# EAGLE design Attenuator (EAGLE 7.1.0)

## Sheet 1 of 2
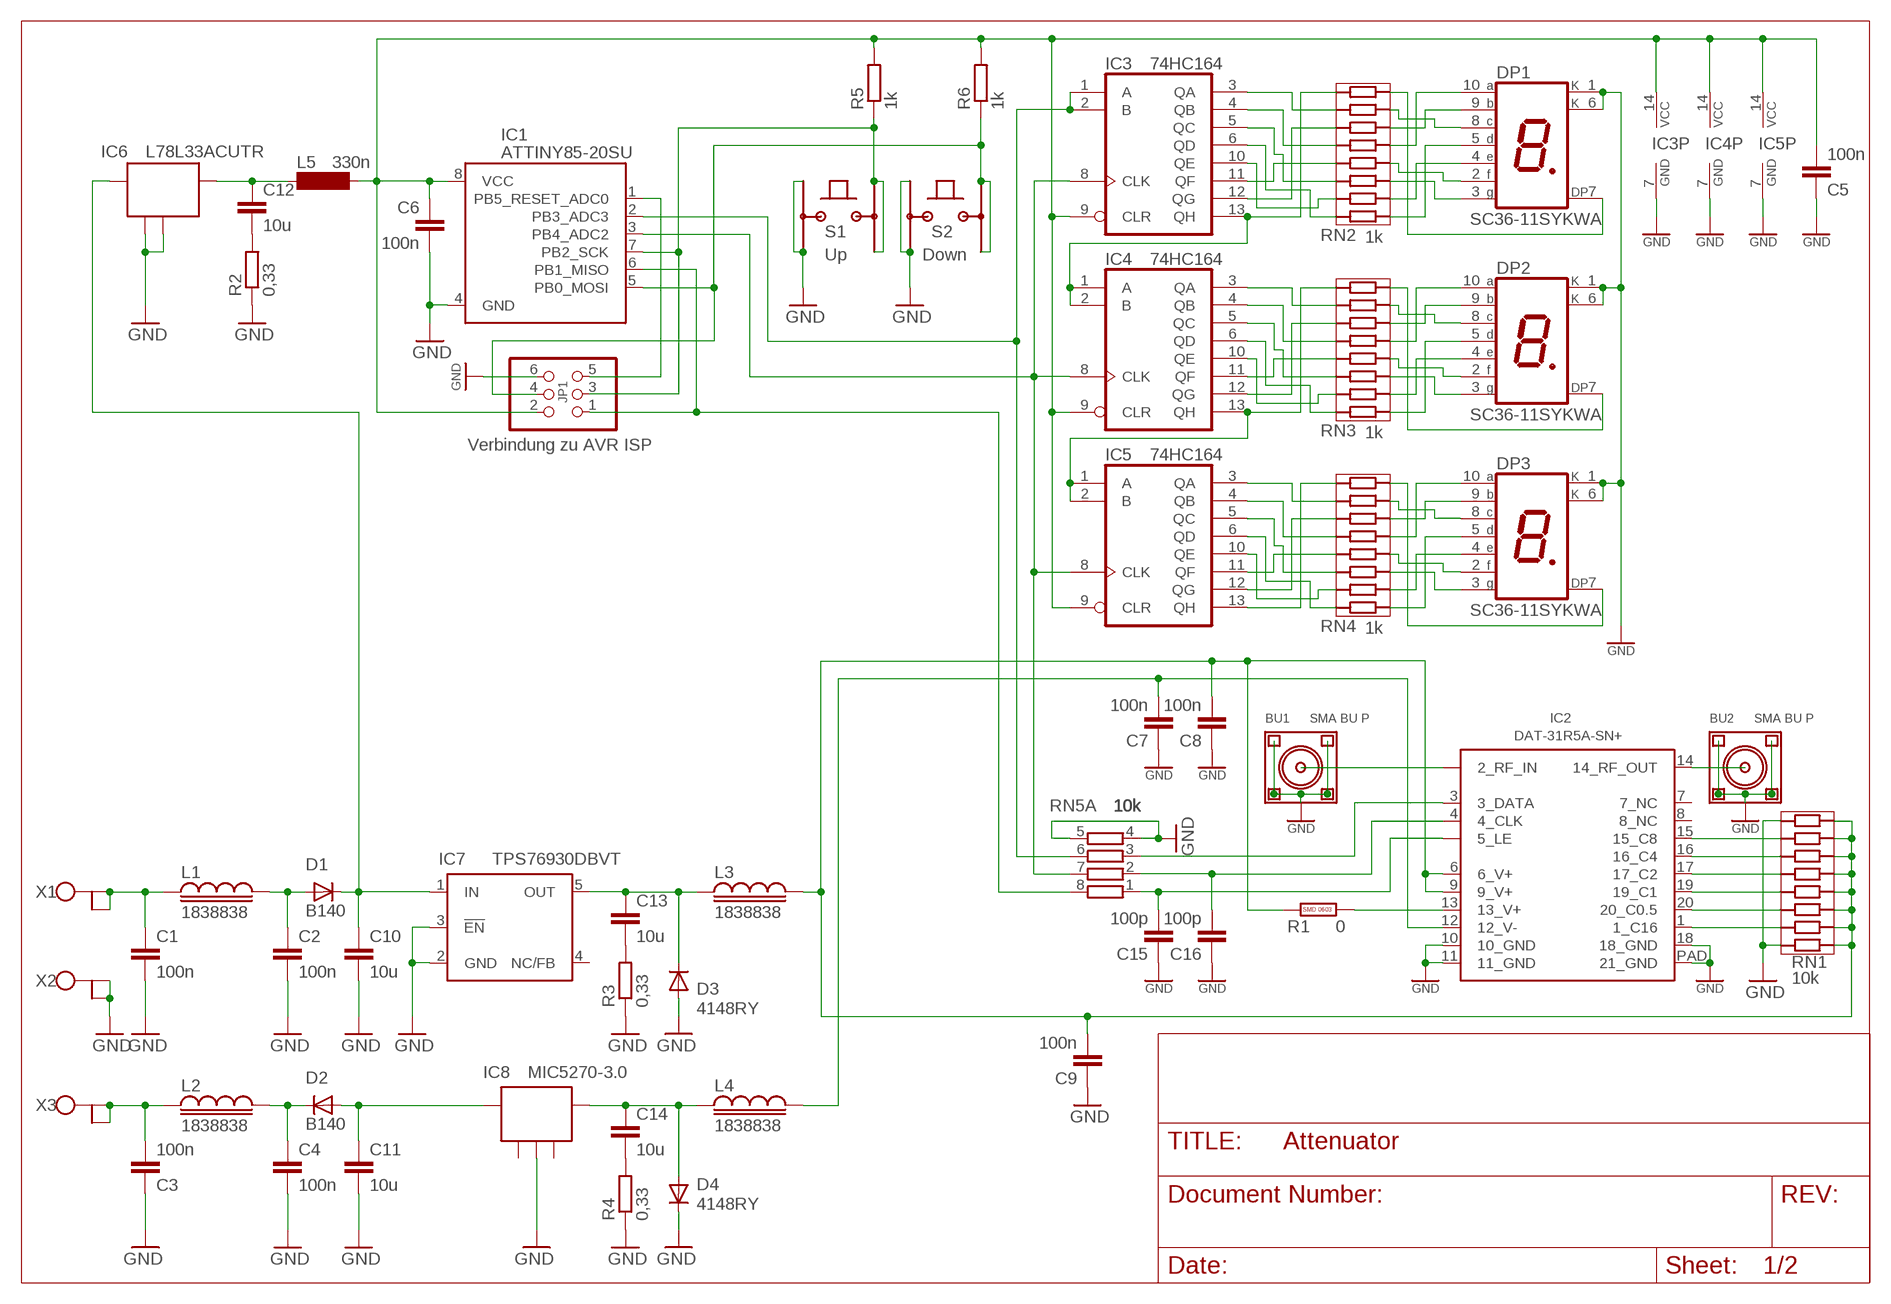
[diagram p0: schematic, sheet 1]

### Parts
BU1  SMA BU P  SMA_BUCHSE_STEHEND  [BU_SMA_STEHEND]
BU2  SMA BU P  SMA_BUCHSE_STEHEND  [BU_SMA_STEHEND]
C1  100n  C-EUC0805  [C0805]
C2  100n  C-EUC0805  [C0805]
C3  100n  C-EUC0805  [C0805]
C4  100n  C-EUC0805  [C0805]
C5  100n  C-EUC0805  [C0805]
C6  100n  C-EUC1206  [C1206]
C7  100n  C-EUC0603K  [C0603K]
C8  100n  C-EUC0603K  [C0603K]
C9  100n  C-EUC0603K  [C0603K]
C10  10u  C-EUC0805  [C0805]
C11  10u  C-EUC0805  [C0805]
C12  10u  C-EUC0805  [C0805]
C13  10u  C-EUC0805  [C0805]
C14  10u  C-EUC0805  [C0805]
C15  100p  C-EUC0603K  [C0603K]
C16  100p  C-EUC0603K  [C0603K]
D1  B140  DIODE-DO214AC  [DO214AC]
D2  B140  DIODE-DO214AC  [DO214AC]
D3  4148RY  TS4148_0805  [DIODE_0805]
D4  4148RY  TS4148_0805  [DIODE_0805]
DP1  SC36-11SYKWA  SC36-11SWRA_ROUND  [SC36-11SWRA_ROUND]
DP2  SC36-11SYKWA  SC36-11SWRA_ROUND  [SC36-11SWRA_ROUND]
DP3  SC36-11SYKWA  SC36-11SWRA_ROUND  [SC36-11SWRA_ROUND]
IC1  ATTINY85-20SU  [8S2]
IC2  DAT-31R5A-SN+  DAT-31-PP  [DG983-1]
IC3  74HC164  74AC164D  [SO14]
IC4  74HC164  74AC164D  [SO14]
IC5  74HC164  74AC164D  [SO14]
IC6  L78L33ACUTR  78XX_SOT89  [SOT89]
IC7  TPS76930DBVT  TPS77001  [SOT23-DBV]
IC8  MIC5270-3.0  [SOT23-5]
JP1  Verbindung zu AVR ISP  PINHD-2X3_2.54-SMD  [2X03SMD]
L1  1838838  L_0805  [SMD_0805]
L2  1838838  L_0805  [SMD_0805]
L3  1838838  L_0805  [SMD_0805]
L4  1838838  L_0805  [SMD_0805]
L5  330n  SM-1206  [SM-1206]
R1  0  MY_R0603  [X0603]
R2  0,33  R-EU_R0805  [R0805]
R3  0,33  R-EU_R0805  [R0805]
R4  0,33  R-EU_R0805  [R0805]
R5  1k  R-EU_R0805  [R0805]
R6  1k  R-EU_R0805  [R0805]
RN1  10k  RN_742C163  [RN_8_0.8MM]
RN2  1k  RN_742C163  [RN_8_0.8MM]
RN3  1k  RN_742C163  [RN_8_0.8MM]
RN4  1k  RN_742C163  [RN_8_0.8MM]
RN5  10k  4R-NEXB38V  [EXB38V]
S1  Up  TASTER9315  [TASTER9315]
S2  Down  TASTER9315  [TASTER9315]
X1  WAGO236-1  [WAGO236-1]
X2  WAGO236-1  [WAGO236-1]
X3  WAGO236-1  [WAGO236-1]

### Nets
+3,3V: C5.2 C6.1 IC1.8(VCC) IC3.9(CLR) IC3.14(VCC) IC4.9(CLR) IC4.14(VCC) IC5.9(CLR) IC5.14(VCC) JP1.2 L5.2 R5.2 R6.2
+3V: C8.2 C9.2 IC2.6(6_V+) IC2.9(9_V+) L3.2 R1.2 RN1.1 RN1.2 RN1.3 RN1.4 RN1.5 RN1.6 RN1.7 RN1.8
-3V: C7.2 IC2.12(12_V-) L4.2
CLK: IC1.3(PB4_ADC2) IC3.8(CLK) IC4.8(CLK) IC5.8(CLK) RN5.7
DATA: IC1.2(PB3_ADC3) IC3.1(A) IC3.2(B) RN5.6
GND: BU1.GND BU1.GND@1(GND) BU1.GND@2(GND) BU1.GND@3(GND) BU2.GND BU2.GND@1(GND) BU2.GND@2(GND) BU2.GND@3(GND) C1.2 C2.2 C3.1 C4.2 C5.1 C6.2 C7.1 C8.1 C9.1 C10.2 C11.2 C15.1 C16.1 D3.A D4.K(C) DP1.1(A) DP1.6(A) DP2.1(A) DP2.6(A) DP3.1(A) DP3.6(A) IC1.4(GND) IC2.10(10_GND) IC2.11(11_GND) IC2.18(18_GND) IC2.PAD(21_GND) IC3.7(GND) IC4.7(GND) IC5.7(GND) IC6.2(GND) IC6.2@1(CASE) IC7.2(GND) IC7.3(!EN) IC8.2(GND) JP1.6 R2.1 R3.1 R4.1 RN1.9 RN1.16 RN5.4 RN5.5 S1.1 S1.2 S2.1 S2.2 X2.1(KL) X2.2(KL1) ; also sheet 2
MISO: IC1.6(PB1_MISO) JP1.1 RN5.8
MOSI: IC1.5(PB0_MOSI) JP1.4 R6.1 S2.3 S2.4
N$1: IC2.3(3_DATA) RN5.3
N$2: C10.1 D1.C IC6.3(OUT) IC7.1(IN)
N$3: C1.1 L1.1 X1.1(KL) X1.2(KL1)
N$4: C12.2 R2.2
N$5: C2.1 D1.A L1.2
N$6: IC2.1(1_C16) RN1.10
N$7: C13.2 R3.2
N$9: IC2.20(20_C0.5) RN1.11
N$10: IC2.19(19_C1) RN1.12
N$11: IC2.17(17_C2) RN1.13
N$12: IC2.16(16_C4) RN1.14
N$13: IC2.15(15_C8) RN1.15
N$14: C16.2 IC2.4(4_CLK) RN5.2
N$15: C15.2 IC2.5(5_LE) RN5.1
N$16: IC2.13(13_V+) R1.1
N$19: C13.1 D3.K(C) IC7.5(OUT) L3.1
N$59: C14.2 R4.2
N$60: C12.1 IC6.1(IN) L5.1
N$61: C3.2 L2.1 X3.1(KL) X3.2(KL1)
N$62: C4.1 D2.C L2.2
N$63: C11.1 D2.A IC8.5(-IN)
N$64: C14.1 D4.A IC8.4(-OUT) L4.1
N$73: DP2.7(DP) RN3.16
N$80: DP2.8(C) RN3.15
N$81: DP2.9(B) RN3.14
N$82: DP2.10(A) RN3.13
N$83: DP2.2(F) RN3.12
N$84: DP2.3(G) RN3.11
N$85: DP2.4(E) RN3.10
N$86: DP2.5(D) RN3.9
N$87: DP1.7(DP) RN2.16
N$88: IC4.13(QH) IC5.1(A) IC5.2(B) RN3.1
N$89: IC4.5(QC) RN3.6
N$90: IC4.3(QA) RN3.2
N$91: IC4.12(QG) RN3.3
N$92: IC4.4(QB) RN3.4
N$93: IC4.11(QF) RN3.5
N$94: IC4.10(QE) RN3.7
N$96: IC4.6(QD) RN3.8
N$97: DP1.8(C) RN2.15
N$98: DP1.9(B) RN2.14
N$99: DP1.10(A) RN2.13
N$100: DP1.2(F) RN2.12
N$101: DP1.3(G) RN2.11
N$102: DP1.4(E) RN2.10
N$103: DP1.5(D) RN2.9
N$105: IC3.13(QH) IC4.1(A) IC4.2(B) RN2.1
N$106: IC3.3(QA) RN2.2
N$107: IC3.12(QG) RN2.3
N$108: IC3.4(QB) RN2.4
N$109: IC3.11(QF) RN2.5
N$110: IC3.5(QC) RN2.6
N$111: IC3.10(QE) RN2.7
N$112: IC3.6(QD) RN2.8
N$113: DP3.7(DP) RN4.16
N$114: DP3.8(C) RN4.15
N$115: DP3.9(B) RN4.14
N$116: DP3.10(A) RN4.13
N$117: DP3.2(F) RN4.12
N$118: DP3.3(G) RN4.11
N$119: DP3.4(E) RN4.10
N$120: DP3.5(D) RN4.9
N$122: IC5.13(QH) RN4.1
N$123: IC5.3(QA) RN4.2
N$124: IC5.12(QG) RN4.3
N$125: IC5.4(QB) RN4.4
N$126: IC5.11(QF) RN4.5
N$127: IC5.5(QC) RN4.6
N$128: IC5.10(QE) RN4.7
N$129: IC5.6(QD) RN4.8
RESET1: IC1.1(PB5_RESET_ADC0) JP1.5
RF_IN: BU1.SIGNAL IC2.2(2_RF_IN)
RF_OUT: BU2.SIGNAL IC2.14(14_RF_OUT)
SCK: IC1.7(PB2_SCK) JP1.3 R5.1 S1.3 S1.4
Unconnected: IC2.7(7_NC) IC2.8(8_NC) IC7.4(NC/FB) IC8.1(NC1) IC8.3(NC2)

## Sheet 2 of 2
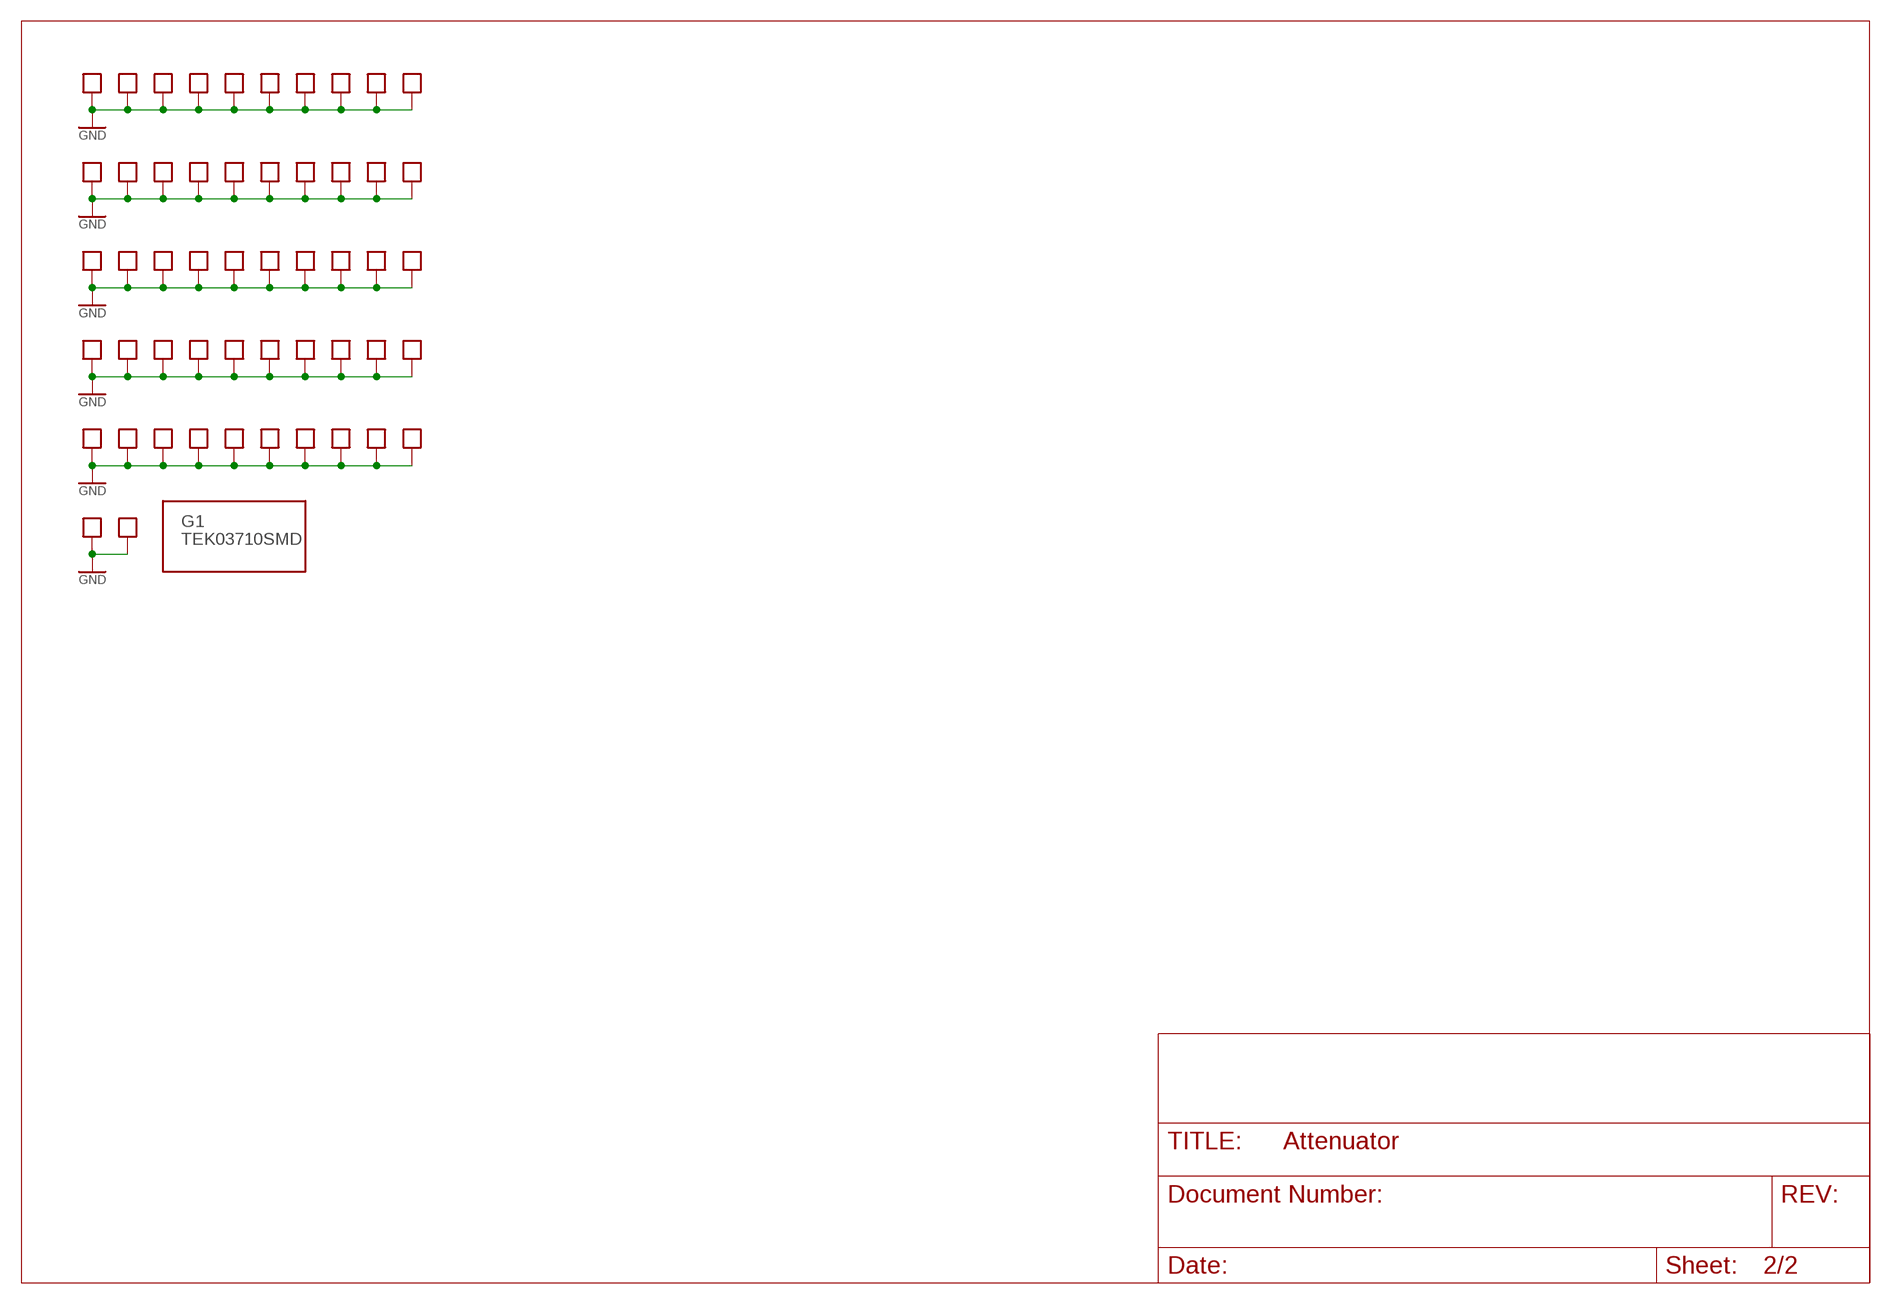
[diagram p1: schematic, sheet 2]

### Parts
G1  TEK03710SMD  [TEKO3710SMD]
GP1  PAD_1X1.5  [PAD_254X381]
GP2  PAD_1X1.5  [PAD_254X381]
GP3  PAD_1X1.5  [PAD_254X381]
GP4  PAD_1X1.5  [PAD_254X381]
GP5  PAD_1X1.5  [PAD_254X381]
GP6  PAD_1X1.5  [PAD_254X381]
GP7  PAD_1X1.5  [PAD_254X381]
GP8  PAD_1X1.5  [PAD_254X381]
GP9  PAD_1X1.5  [PAD_254X381]
GP10  PAD_1X1.5  [PAD_254X381]
GP11  PAD_1X1.5  [PAD_254X381]
GP12  PAD_1X1.5  [PAD_254X381]
GP13  PAD_1X1.5  [PAD_254X381]
GP14  PAD_1X1.5  [PAD_254X381]
GP15  PAD_1X1.5  [PAD_254X381]
GP16  PAD_1X1.5  [PAD_254X381]
GP17  PAD_1X1.5  [PAD_254X381]
GP18  PAD_1X1.5  [PAD_254X381]
GP19  PAD_1X1.5  [PAD_254X381]
GP20  PAD_1X1.5  [PAD_254X381]
GP21  PAD_1X1.5  [PAD_254X381]
GP22  PAD_1X1.5  [PAD_254X381]
GP23  PAD_1X1.5  [PAD_254X381]
GP24  PAD_1X1.5  [PAD_254X381]
GP25  PAD_1X1.5  [PAD_254X381]
GP26  PAD_1X1.5  [PAD_254X381]
GP27  PAD_1X1.5  [PAD_254X381]
GP28  PAD_1X1.5  [PAD_254X381]
GP29  PAD_1X1.5  [PAD_254X381]
GP30  PAD_1X1.5  [PAD_254X381]
GP31  PAD_1X1.5  [PAD_254X381]
GP32  PAD_1X1.5  [PAD_254X381]
GP33  PAD_1X1.5  [PAD_254X381]
GP34  PAD_1X1.5  [PAD_254X381]
GP35  PAD_1X1.5  [PAD_254X381]
GP36  PAD_1X1.5  [PAD_254X381]
GP37  PAD_1X1.5  [PAD_254X381]
GP38  PAD_1X1.5  [PAD_254X381]
GP39  PAD_1X1.5  [PAD_254X381]
GP40  PAD_1X1.5  [PAD_254X381]
GP41  PAD_1X05  [PAD_254X127]
GP42  PAD_1X1.5  [PAD_254X381]
GP43  PAD_1X1.5  [PAD_254X381]
GP44  PAD_1X1.5  [PAD_254X381]
GP45  PAD_1X1.5  [PAD_254X381]
GP46  PAD_1X1.5  [PAD_254X381]
GP47  PAD_1X1.5  [PAD_254X381]
GP48  PAD_1X1.5  [PAD_254X381]
GP49  PAD_1X1.5  [PAD_254X381]
GP50  PAD_1X1.5  [PAD_254X381]
GP51  PAD_1X1.5  [PAD_254X381]
GP52  PAD_1X05  [PAD_254X127]

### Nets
GND: GP1.TP(GND) GP2.TP(GND) GP3.TP(GND) GP4.TP(GND) GP5.TP(GND) GP6.TP(GND) GP7.TP(GND) GP8.TP(GND) GP9.TP(GND) GP10.TP(GND) GP11.TP(GND) GP12.TP(GND) GP13.TP(GND) GP14.TP(GND) GP15.TP(GND) GP16.TP(GND) GP17.TP(GND) GP18.TP(GND) GP19.TP(GND) GP20.TP(GND) GP21.TP(GND) GP22.TP(GND) GP23.TP(GND) GP24.TP(GND) GP25.TP(GND) GP26.TP(GND) GP27.TP(GND) GP28.TP(GND) GP29.TP(GND) GP30.TP(GND) GP31.TP(GND) GP32.TP(GND) GP33.TP(GND) GP34.TP(GND) GP35.TP(GND) GP36.TP(GND) GP37.TP(GND) GP38.TP(GND) GP39.TP(GND) GP40.TP(GND) GP41.TP(GND) GP42.TP(GND) GP43.TP(GND) GP44.TP(GND) GP45.TP(GND) GP46.TP(GND) GP47.TP(GND) GP48.TP(GND) GP49.TP(GND) GP50.TP(GND) GP51.TP(GND) GP52.TP(GND) ; also sheet 1

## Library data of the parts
BU1 BU2 = Diverse Analog:SMA_BUCHSE_STEHEND
C1-C16 = rcl:C-EU: CAPACITOR, European symbol
D1 D2 = diode:DIODE-: DIODE
D3 D4 = Dioden:TS4148_0805
DP1-DP3 = Displays:SC36-11SWRA_ROUND
G1 = Diverse Analog:TEK03710SMD
GP1-GP40 GP42-GP51 = Diverse Analog:PAD_1X1.5
GP41 GP52 = Diverse Analog:PAD_1X05
IC1 = Diverse Analog:ATTINY85-20SU
IC2 = Diverse Analog:DAT-31-PP
IC3-IC5 = 74xx-eu:74*164: 8-bit parallel out SHIFT REGISTER
IC6 = Diverse Analog:78XX_SOT89
IC7 = texas:TPS770*: ULTRALOW-POWER 50-mA LOW-DROPOUT LINEAR REGULATORS 50-mA Low-Dropout Regulator Source: http://focus.ti.com/lit/ds/symlink/tps77001.pdf
IC8 = Diverse Analog:MIC5270-3.0
JP1 = pinhead1:PINHD-2X3: PIN HEADER
L1-L4 = Diverse Analog:L_0805
L5 = inductor-neosid:SM-1206: INDUCTOR
R1 = Diverse Analog:MY_R0603
R2-R6 = rcl:R-EU_: RESISTOR, European symbol
RN1-RN4 = Diverse Analog:RN_742C163
RN5 = resistor-dil:4R-N: Array Chip Resistor Source: RS Component / Phycomp
S1 S2 = Diverse Analog:TASTER9315
X1-X3 = Diverse Analog:WAGO236-1

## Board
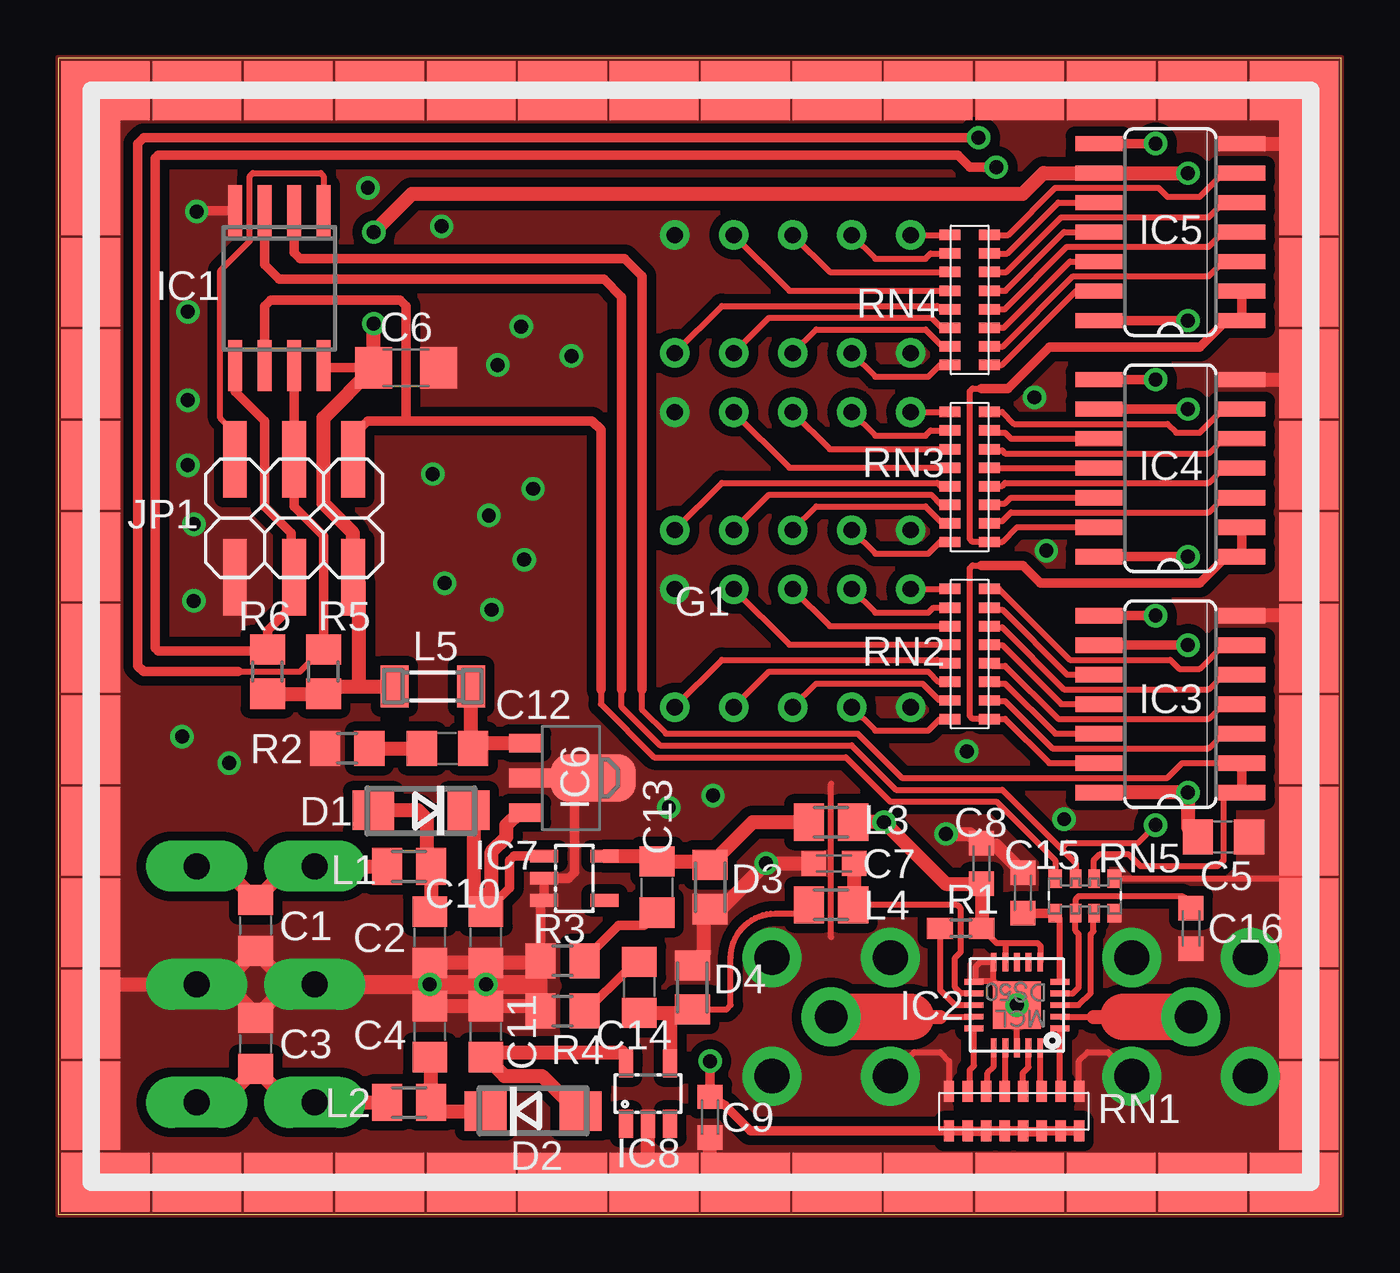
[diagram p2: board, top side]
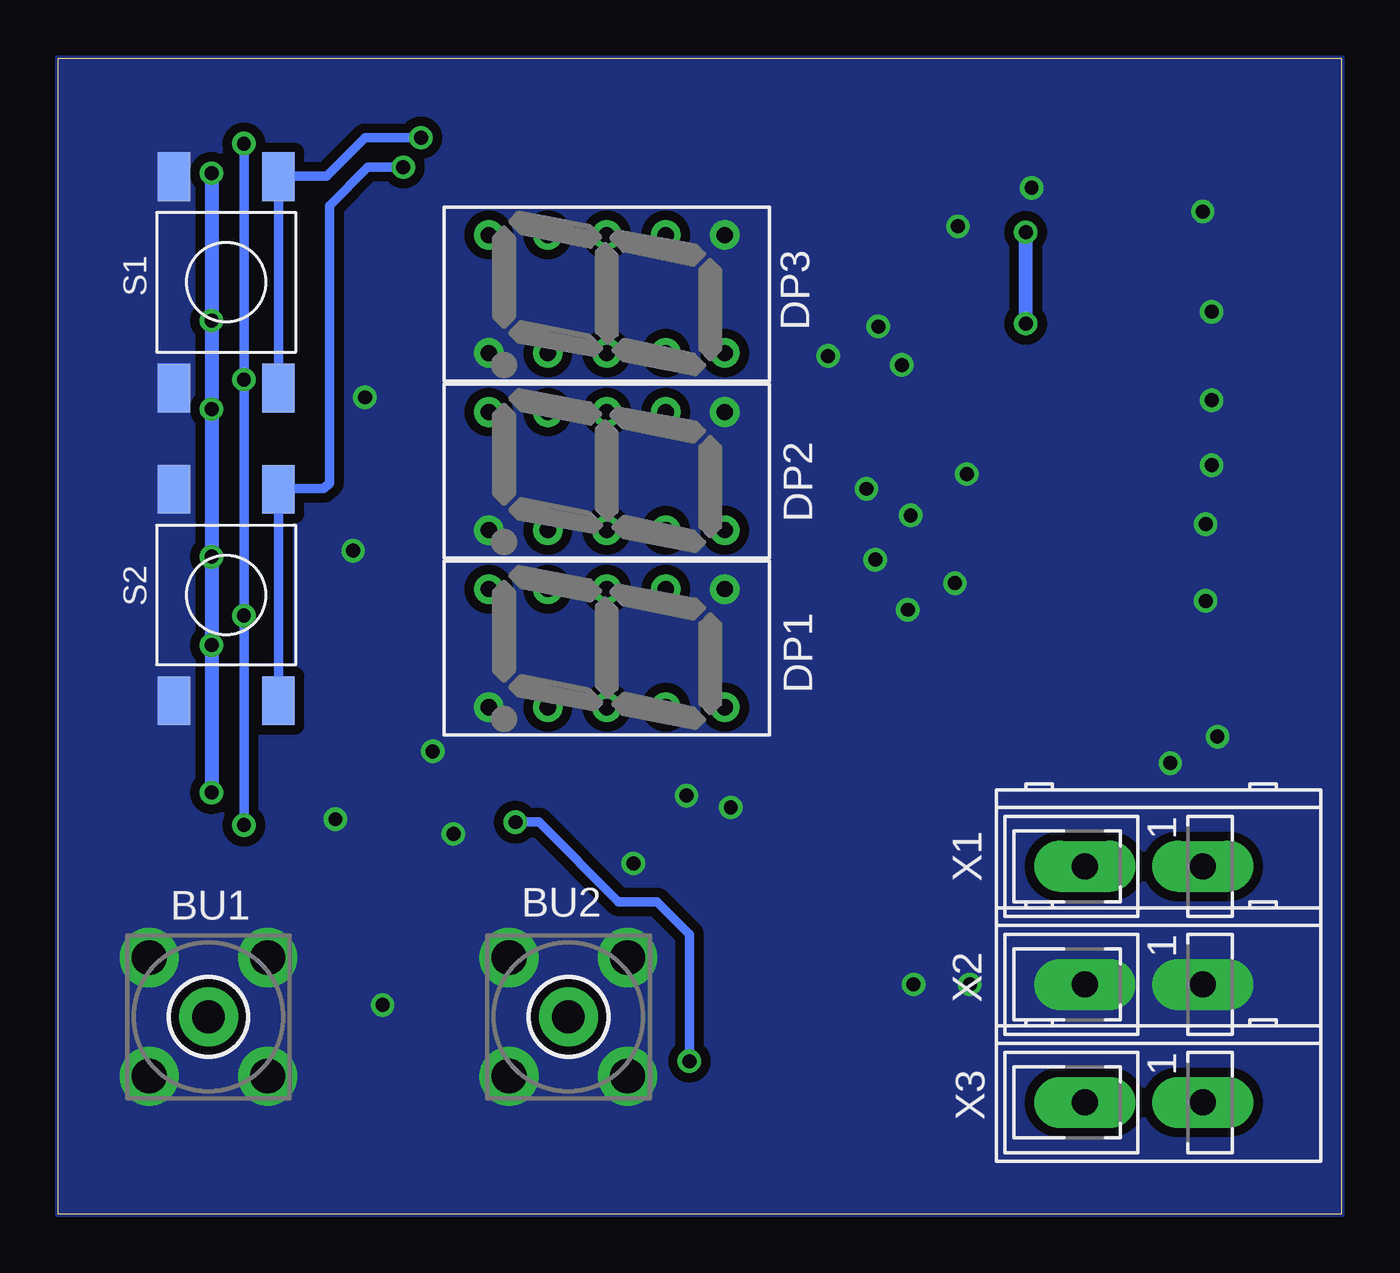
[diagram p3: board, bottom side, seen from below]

Size 55.24 x 49.78 mm. Coordinates in mm from the lower left corner, seen from the top.
Outline: 0,0 55.24,0 55.24,49.78 0,49.78 0,0
Copper layers (1*16): Top 0.035mm / dielectric 1.5mm / Bottom 0.035mm
Design rules "default *": minimum track width 10mil, minimum drill 24mil, track to track 6mil, track to pad 6mil, pad to pad 6mil, via to via 6mil, smd to smd 6mil, copper to edge 0mil, drill to drill 8mil, minimum pad ring 10mil, minimum via ring 8mil, stop-mask expansion 4mil, vias tented up to drill 0mil, thermal gap 10mil

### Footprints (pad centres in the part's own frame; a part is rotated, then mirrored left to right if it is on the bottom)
BU_SMA_STEHEND = drill 1.5 pad 2.54: GND 2.55,2.55; GND@1 -2.55,2.55; GND@2 -2.55,-2.55; GND@3 2.55,-2.55 | drill 1.4 pad 2.54: SIGNAL 0,0
C0805 = smd 1.3 x 1.5: 1 -1.1,0; 2 1.1,0
C1206 = smd 1.6 x 1.8: 1 -1.4,0; 2 1.4,0
C0603K = smd 1.05 x 1.08: 1 -0.875,0; 2 0.875,0
DO214AC = smd 1.8 x 1.7: A 2.05,0; C -2.05,0
DIODE_0805 = smd 1.3 x 1.5: A 0.95,0; K -0.95,0
SC36-11SWRA_ROUND = drill 0.7 pad 1.27: 1 -2.54,5.08; 2 -2.54,2.54; 3 -2.54,0; 4 -2.54,-2.54; 5 -2.54,-5.08; 6 2.54,-5.08; 7 2.54,-2.54; 8 2.54,0; 9 2.54,2.54; 10 2.54,5.08
PAD_254X381 = smd 3.81 x 2.54: TP 0,0
PAD_254X127 = smd 1.27 x 2.54: TP 0,0
8S2 = smd 0.6 x 2.2: 1 -1.905,-3.337; 2 -0.635,-3.337; 3 0.635,-3.337; 4 1.905,-3.337; 5 1.905,3.337; 6 0.635,3.337; 7 -0.635,3.337; 8 -1.905,3.337
DG983-1 = smd 0.81 x 0.25: 1 -1.845,1; 2 -1.845,0.5; 3 -1.845,0; 4 -1.845,-0.5; 5 -1.845,-1; 11 1.845,-1; 12 1.845,-0.5; 13 1.845,0; 14 1.845,0.5; 15 1.845,1 | smd 0.25 x 0.81: 6 -1,-1.845; 7 -0.5,-1.845; 8 0,-1.845; 9 0.5,-1.845; 10 1,-1.845; 16 1,1.845; 17 0.5,1.845; 18 0,1.845; 19 -0.5,1.845; 20 -1,1.845 | smd 2.06 x 2.06: PAD 0,0
SO14 = smd 0.66 x 2.032: 1 -3.81,-3.073; 2 -2.54,-3.073; 3 -1.27,-3.073; 4 0,-3.073; 5 1.27,-3.073; 6 2.54,-3.073; 7 3.81,-3.073; 8 3.81,3.073; 9 2.54,3.073; 10 1.27,3.073; 11 0,3.073; 12 -1.27,3.073; 13 -2.54,3.073; 14 -3.81,3.073
SOT89 = smd 0.8 x 1.4: 1 -1.499,-1.981; 3 1.499,-1.981 | smd 0.8 x 1.9: 2 0,-1.727 | smd 2.032 x 3.65: 2@1 0,0.94
SOT23-DBV = smd 0.55 x 1.2: 1 -0.95,-1.3; 2 0,-1.3; 3 0.95,-1.3; 4 0.95,1.3; 5 -0.95,1.3
SOT23-5 = smd 0.6 x 1.2: 1 -0.95,-1.3; 2 0,-1.3; 3 0.95,-1.3; 4 0.95,1.3; 5 -0.95,1.3
2X03SMD = smd 1.016 x 3.302: 1 -1.27,-3.81; 2 -1.27,1.27; 3 1.27,-3.81; 4 1.27,1.27; 5 3.81,-3.81; 6 3.81,1.27
SMD_0805 = smd 1.3 x 1.6: 1 -0.95,0; 2 0.95,0
SM-1206 = smd 1.2 x 1.8: 1 -1.65,0; 2 1.65,0
X0603 = smd 1.1 x 0.9: 1 -0.9,0; 2 0.9,0
R0805 = smd 1.3 x 1.5: 1 -0.95,0; 2 0.95,0
RN_8_0.8MM = smd 0.45 x 0.9: 1 -2.8,-0.85; 2 -2,-0.85; 3 -1.2,-0.85; 4 -0.4,-0.85; 5 0.4,-0.85; 6 1.2,-0.85; 7 2,-0.85; 8 2.8,-0.85; 9 2.8,0.85; 10 2,0.85; 11 1.2,0.85; 12 0.4,0.85; 13 -0.4,0.85; 14 -1.2,0.85; 15 -2,0.85; 16 -2.8,0.85
EXB38V = smd 0.6 x 0.8: 1 -1.275,-0.75; 4 1.275,-0.75; 5 1.275,0.75; 8 -1.275,0.75 | smd 0.5 x 0.8: 2 -0.4,-0.75; 3 0.4,-0.75; 6 0.4,0.75; 7 -0.4,0.75
TASTER9315 = smd 2.1 x 1.4: 1 4.55,-2.25; 2 -4.55,-2.25; 3 4.55,2.25; 4 -4.55,2.25
WAGO236-1 = drill 1.118 pad 2.184 long: 1 0,-2.54; 2 0,2.54

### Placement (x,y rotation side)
BU1  48.77,8.51 0 bottom
BU2  33.27,8.51 0 bottom
C1  8.51,12.45 270 top
C2  16,11.94 270 top
C3  8.51,7.37 270 top
C4  16,7.87 90 top
C5  50.16,16.26 180 top
C6  14.99,36.45 0 top
C7  33.4,15.11 0 top
C8  39.75,15.11 270 top
C9  28.07,4.19 90 top
C10  18.41,11.94 270 top
C11  18.41,7.87 90 top
C12  16.76,20.07 180 top
C13  25.78,14.1 270 top
C14  25.02,9.78 90 top
C15  41.53,13.84 270 top
C16  48.77,12.32 90 top
D1  15.62,17.4 180 top
D2  20.45,4.45 0 top
D3  28.07,14.1 270 top
D4  27.3,9.78 270 top
DP1  31.62,24.38 270 bottom
DP2  31.62,32 270 bottom
DP3  31.62,39.62 270 bottom
G1  27.69,24.89 0 top
GP1  2.03,1.4 0 top
GP2  5.97,1.4 0 top
GP3  9.91,1.4 0 top
GP4  1.4,4.7 90 top
GP5  13.84,1.4 0 top
GP6  17.78,1.4 0 top
GP7  21.72,1.4 0 top
GP8  25.65,1.4 0 top
GP9  29.59,1.4 0 top
GP10  33.53,1.4 0 top
GP11  53.85,44.07 90 top
GP12  37.47,1.4 180 top
GP13  53.21,48.39 180 top
GP14  41.4,1.4 180 top
GP15  49.28,48.39 180 top
GP16  45.34,1.4 180 top
GP17  45.34,48.39 180 top
GP18  49.28,1.4 180 top
GP19  41.4,48.39 180 top
GP20  53.21,1.4 180 top
GP21  37.47,48.39 180 top
GP22  53.85,4.7 90 top
GP23  33.53,48.39 180 top
GP24  53.85,8.64 90 top
GP25  29.59,48.39 180 top
GP26  53.85,12.57 90 top
GP27  25.65,48.39 180 top
GP28  53.85,16.51 90 top
GP29  21.72,48.39 180 top
GP30  53.85,20.45 90 top
GP31  17.78,48.39 180 top
GP32  53.85,24.38 90 top
GP33  13.84,48.39 180 top
GP34  53.85,28.32 90 top
GP35  9.91,48.39 180 top
GP36  53.85,32.26 90 top
GP37  5.97,48.39 180 top
GP38  53.85,36.2 90 top
GP39  2.03,48.39 180 top
GP40  53.85,40.13 90 top
GP41  53.85,46.61 90 top
GP42  1.4,24.38 90 top
GP43  1.4,44.07 90 top
GP44  1.4,20.45 90 top
GP45  1.4,40.13 90 top
GP46  1.4,16.51 90 top
GP47  1.4,36.2 90 top
GP48  1.4,12.57 90 top
GP49  1.4,32.26 90 top
GP50  1.4,8.64 90 top
GP51  1.4,28.32 90 top
GP52  1.4,46.48 90 top
IC1  9.53,39.88 180 top
IC2  41.27,9.02 180 top
IC3  47.88,21.97 90 top
IC4  47.88,32.13 90 top
IC5  47.88,42.29 90 top
IC6  22.1,18.8 270 top
IC7  22.23,14.48 270 top
IC8  25.4,5.21 0 top
JP1  11.43,28.7 180 top
L1  15.11,14.99 0 top
L2  15.11,4.83 0 top
L3  33.27,16.89 0 top
L4  33.27,13.34 0 top
L5  16.13,22.73 180 top
R1  38.86,12.32 0 top
R2  12.45,20.07 0 top
R3  21.72,10.92 0 top
R4  21.72,8.76 0 top
R5  11.43,23.37 270 top
R6  9.02,23.37 270 top
RN1  41.15,4.45 0 top
RN2  39.24,24.13 90 top
RN3  39.24,31.75 90 top
RN4  39.24,39.37 90 top
RN5  44.2,13.72 0 top
S1  48.01,40.13 270 bottom
S2  48.01,26.67 270 bottom
X1  8.51,14.99 270 bottom
X2  8.51,9.91 270 bottom
X3  8.51,4.83 270 bottom

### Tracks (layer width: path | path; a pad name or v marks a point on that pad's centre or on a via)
+3,3V  (via drill 0.6)
  Top 0.406: C6.1 11.52,36.45 IC1.8 | R5.2 11.74,22.73 | v48.64,38.48 IC5.14 | v48.64,34.67 IC4.9 | v48.64,28.32 IC4.14 | v48.64,24.51 IC3.9
  Top 0.61: IC3.14 v48.64,18.16 48.64,16.68 C5.2 | v13.59,42.29 15.24,43.94 41.53,43.94 42.42,44.83 IC5.9 v48.64,44.83 | v13.59,38.35 C6.1 11.43,34.29 11.43,30.61 12.7,29.34 JP1.2 12.95,27.18 12.95,22.73 | R6.2 R5.2 | 12.95,22.73 L5.2 | 11.74,22.73 12.95,22.73
  Bottom 0.61: v48.64,44.83 v48.64,38.48 v48.64,34.67 v48.64,28.32 v48.64,24.51 v48.64,18.16 | v13.59,38.35 v13.59,42.29
+3V  (via drill 0.6)
  Top 0.254: IC2.9 40.77,11.68 | 40.77,11.68 42.16,11.68 42.29,11.56 42.29,10.88 IC2.6 | 40.77,11.68 40.4,11.68 R1.2 | RN1.2 39.2,3.6 39.24,3.56 | 39.94,3.56 39.94,3.59 RN1.3 | 40.77,3.56 40.77,3.58 RN1.4 | 42.35,3.56 42.35,3.59 RN1.6
  Top 0.406: RN1.8 RN1.7 RN1.6 | 42.35,3.59 42.29,3.59 42.29,3.56 41.55,3.56 RN1.5 RN1.4 RN1.3 | 39.94,3.59 39.15,3.59 RN1.2 RN1.1 29.81,3.6 28.7,4.7 C9.2 v28.07,6.6
  Top 0.61: R1.2 39.76,14.23 C8.2 38.21,14.24 v35.56,16.89 L3.2
  Bottom 0.406: v35.56,16.89 34.54,16.89 31.11,13.46 29.46,13.46 28.07,12.06 v28.07,6.6
-3V
  Top 0.254: IC2.12 38.87,9.52 38.61,9.78 38.61,11.05 38.86,11.3 38.86,13.08 arc90 38.61,13.34 L4.2
  Top 0.61: C7.2 34.28,13.39 arc-90 L4.2
CLK  (via drill 0.6)
  Top 0.254: 43.18,15.75 40.64,18.29 36.07,18.29 34.16,20.19 25.91,20.19 24.26,21.84 24.26,22.61 | 43.18,15.75 43.81,15.11 43.81,14.48 RN5.7 | 43.18,15.75 43.43,16 46.48,16 v47.24,16.76
  Top 0.406: v47.24,46.1 IC5.8 | v47.24,35.94 IC4.8 | v47.24,25.78 IC3.8 | IC1.3 8.89,40.89 9.53,40.26 23.5,40.26 24.26,39.5 24.26,22.61
  Bottom 0.406: v47.24,16.76 v47.24,25.78 v47.24,35.94 v47.24,46.1
DATA
  Top 0.254: 50.93,18.14 50.19,18.14 arc-90 50.16,18.16 50.16,15.24 49.91,14.99 46.61,14.99 46.1,15.49 44.83,15.49 44.58,15.24 44.58,14.48 RN5.6 | IC3.2 48.39,19.43 47.75,18.8 36.32,18.8 34.42,20.7 26.16,20.7 25.15,21.72 25.15,22.61
  Top 0.406: IC3.2 IC3.1 50.93,18.14 | IC1.2 10.16,41.4 10.41,41.15 24.38,41.15 25.15,40.39 25.15,22.61
GND  (via drill 0.6)
  Top 0.254: IC2.11 39.5,10.08 39.5,10.67 39.69,10.86 IC2.10 40.26,10.85 40.26,10.03 | IC2.18 IC2.PAD 40.26,10.03 | 40.26,10.03 39.5,10.03 | RN1.9 43.95,6.61 44.32,6.99 45.19,6.99 BU1.GND@3 | RN1.16 38.35,6.6 37.97,6.99 36.85,6.99 BU2.GND@2 | RN5.5 53.84,14.47 53.85,14.48 GP26.TP | 33.27,11.94 33.27,18.54
  Top 0.305: 39.15,1.43 39.12,1.4 GP12.TP
  Top 0.406: 22.23,18.67 22.23,14.73 21.97,14.48 IC7.2 IC7.3 20.77,13.37 R3.1 | 22.23,18.67 22.35,18.8 IC6.2@1 | IC6.2 22.1,18.8 22.23,18.67 | IC1.4 6,43.22 v5.97,43.18
  Top 0.61: C7.1 v30.48,15.11 28.57,13.21 28.13,13.21 D3.A 27.81,12.89 27.81,11.3 27.3,10.79 D4.K | C4.2 C11.2 20.56,8.97 R4.1 R3.1 20.68,10.84 C10.2 C2.2 | 7.15,9.99 7.07,9.91 X2.2 1.52,9.91 1.4,10.03 GP50.TP | 7.15,9.99 C1.2 | 9.91,9.91 8.64,11.18 | C3.1 8.51,8.64 7.15,9.99 | 9.91,9.91 X2.1 | 9.91,9.91 8.64,8.64 | IC5.7 53.34,46.1 GP41.TP | IC4.7 53.59,35.94 GP38.TP | IC3.7 53.59,25.78 53.85,25.53 GP32.TP | v38.23,16.38 39.24,16.38 39.75,15.88 40.39,15.88 41.53,14.73 | IC8.2 25.4,1.65 GP8.TP | C9.1 28.07,1.4 GP9.TP
  Top 0.813: X2.1 20.57,9.91
  other vias: 5.84,26.42 18.92,36.58 16,9.91 18.41,9.91 16.13,31.88 18.54,30.1 16.64,27.18 20.45,31.24 20.07,28.19 18.67,26.04 19.94,38.23 22.1,36.96 16.51,42.55 5.59,38.86 5.59,35.05 5.59,32.26 5.84,29.72 41.27,9.02 5.33,20.57 7.37,19.43 26.29,17.53 28.19,18.03 13.34,44.2 42.04,35.18 39.12,19.94 42.55,28.57 43.31,17.02
  pour Top (isolate 0.406, no thermals): 0,0 55.24,0 55.24,49.78 0,49.78
  pour Bottom (isolate 0.406, no thermals): 0,0 55.24,0 55.24,49.78 0,49.78
MISO
  Top 0.254: RN5.8 42.92,15.24 40.39,17.78 35.81,17.78 33.91,19.68 25.65,19.68 23.37,21.97 23.37,22.61
  Top 0.406: IC1.6 8.89,39.12 9.14,39.37 14.73,39.37 14.99,39.12 14.99,34.16 | 14.99,34.16 13.34,34.16 12.7,33.53 JP1.1 | 14.99,34.16 22.99,34.16 23.37,33.78 23.37,22.61
MOSI  (via drill 0.6)
  Top 0.406: IC1.5 7.62,35.43 8.89,34.16 8.89,30.48 10.03,29.34 10.03,27.56 JP1.4 10.16,26.29 9.02,25.15 R6.1 8.96,24.26 4.32,24.26 4.19,24.38 4.19,45.47 4.32,45.59 38.73,45.59 39.24,45.09 v40.39,45.09
  Bottom 0.406: v40.39,45.09 41.91,45.09 43.56,43.43 43.56,31.5 43.81,31.24 45.73,31.24 S2.4 S2.3
N$1
  Top 0.254: IC2.3 43.94,9.02 44.45,9.53 44.45,12.06 44.58,12.19 44.58,12.95 RN5.3
N$2
  Top 0.406: IC7.1 19.62,15.43 19.43,15.24 19.43,14.05 C10.1 18.16,13.29 18.16,13.46
  Top 0.61: D1.C 17.91,17.4 17.91,13.55 C10.1 | IC6.3 19.84,17.3 19.3,16.76 19.3,16.26 18.67,15.62 18.67,13.97 18.16,13.46
N$3
  Top 0.61: X1.2 7.07,14.99 C1.1 9.95,14.99 X1.1 L1.1
N$4
  Top 0.61: R2.2 C12.2
N$5
  Top 0.61: C2.1 16.06,13.1 L1.2 15.88,15.17 15.88,17.02 15.49,17.4 D1.A
N$6
  Top 0.254: IC2.1 43.12,5.32 RN1.10
N$7
  Top 0.406: R3.2 22.67,10.98 24.13,12.45 25.23,12.45 C13.2
N$9
  Top 0.254: IC2.20 42.27,5.37 RN1.11
N$10
  Top 0.254: IC2.19 41.77,6.34 41.53,6.1 41.53,5.31 RN1.12
N$11
  Top 0.254: IC2.17 40.77,5.32 RN1.13
N$12
  Top 0.254: IC2.16 40.27,6.37 40.01,6.1 40.01,5.35 RN1.14
N$13
  Top 0.254: IC2.15 39.43,6.41 39.24,6.22 39.24,5.39 RN1.15
N$14
  Top 0.254: C16.2 arc90 48.25,13.72 43.94,13.72 43.81,13.59 43.81,12.98 RN5.2 43.8,12.21 43.94,12.06 43.94,9.78 43.68,9.52 IC2.4
N$15
  Top 0.254: IC2.5 43.12,12.77 RN5.1
  Top 0.406: C15.2 RN5.1 arc-90 RN5.1
N$16
  Top 0.254: IC2.13 38.61,9.02 37.97,9.65 37.97,12.31 R1.1
N$19
  Top 0.61: IC7.5 25.55,15.43 C13.1 27.92,15.2 D3.K 29.91,16.89 L3.1
N$59
  Top 0.406: R4.2 22.73,8.76 24.51,10.54 24.68,10.54 C14.2
N$60
  Top 0.61: IC6.1 18.09,20.3 C12.1 17.78,20.15 L5.1
N$61
  Top 0.61: X3.2 7.07,4.83 C3.2 9.95,4.83 X3.1 L2.1
N$62
  Top 0.61: D2.C 16.44,4.45 L2.2 16.06,6.71 C4.1
N$63
  Top 0.61: D2.A 22.35,4.45 20.83,5.97 19.22,5.97 C11.1 18.63,6.99 24.26,6.99 24.45,6.79 IC8.5
N$64
  Top 0.254: D4.A 28.77,8.83 28.96,9.02 28.96,11.05 arc-90 30.86,12.95 31.94,12.95 L4.1
  Top 0.61: C14.1 26.42,8.68 | 26.42,8.68 27.16,8.68 D4.A | IC8.4 26.35,8.61 26.42,8.68
N$73
  Top 0.254: RN3.16 37.97,28.95 37.47,28.45 35.18,28.45 DP2.7
N$80
  Top 0.254: RN3.15 38.07,29.75 37.34,30.48 32.64,30.48 DP2.8
N$81
  Top 0.254: RN3.14 38.03,30.55 37.59,30.99 30.61,30.99 DP2.9
N$82
  Top 0.254: RN3.13 37.99,31.35 37.85,31.5 28.57,31.5 DP2.10
N$83
  Top 0.254: RN3.12 31.48,32.15 DP2.2
N$84
  Top 0.254: RN3.11 33.22,32.95 DP2.3
N$85
  Top 0.254: RN3.10 37.56,33.75 37.34,33.53 35.18,33.53 DP2.4
N$86
  Top 0.254: RN3.9 DP2.5
N$87
  Top 0.254: RN2.16 37.97,21.33 37.47,20.83 35.18,20.83 DP1.7
N$88
  Top 0.254: IC4.13 41.27,29.59 40.64,28.96 RN3.1 39.37,28.96 39.24,29.08 39.24,35.43 39.37,35.56 39.75,35.56
  Top 0.406: IC5.2 IC5.1 50.29,38.48 49.15,37.34 42.67,37.34 40.89,35.56 39.75,35.56
N$89
  Top 0.254: IC4.5 50.16,33.4 49.53,32.77 40.77,32.77 40.64,32.89 40.15,32.89 RN3.6
N$90
  Top 0.254: IC4.3 50.16,30.86 49.53,30.23 41.02,30.23 40.64,29.84 40.19,29.84 RN3.2
N$91
  Top 0.254: IC4.12 41.02,30.86 40.77,30.61 40.15,30.61 RN3.3
N$92
  Top 0.254: IC4.4 50.16,32.13 49.53,31.5 40.77,31.5 40.64,31.37 40.11,31.37 RN3.4
N$93
  Top 0.254: IC4.11 40.11,32.13 RN3.5
N$94
  Top 0.254: IC4.10 41.02,33.4 40.77,33.66 40.19,33.66 RN3.7
N$96
  Top 0.254: IC4.6 50.16,34.67 49.15,33.66 48.13,33.66 47.75,34.04 41.15,34.04 40.64,34.54 RN3.8
N$97
  Top 0.254: RN2.15 37.94,22.13 37.21,22.86 32.64,22.86 DP1.8
N$98
  Top 0.254: RN2.14 37.9,22.93 37.47,23.37 30.61,23.37 DP1.9
N$99
  Top 0.254: RN2.13 37.99,23.73 37.85,23.88 28.57,23.88 DP1.10
N$100
  Top 0.254: RN2.12 31.48,24.53 DP1.2
N$101
  Top 0.254: RN2.11 33.22,25.33 DP1.3
N$102
  Top 0.254: RN2.10 37.69,26.13 37.47,25.91 35.18,25.91 DP1.4
N$103
  Top 0.254: RN2.9 DP1.5
N$105
  Top 0.254: IC3.13 42.67,19.43 40.77,21.34 RN2.1 39.37,21.34 39.24,21.46 39.24,27.81 39.37,27.94 39.75,27.94
  Top 0.406: 39.75,27.94 41.53,27.94 42.29,27.18 49.15,27.18 50.29,28.32 IC4.1 IC4.2
N$106
  Top 0.254: IC3.3 50.16,20.7 49.53,20.07 42.8,20.07 40.77,22.1 40.12,22.1 RN2.2
N$107
  Top 0.254: RN2.3 40.16,22.86 40.77,22.86 42.93,20.7 IC3.12
N$108
  Top 0.254: IC3.4 50.16,21.97 49.53,21.34 43.05,21.34 40.77,23.62 40.2,23.62 RN2.4
N$109
  Top 0.254: RN2.5 40.11,24.51 40.64,24.51 43.18,21.97 IC3.11
N$110
  Top 0.254: IC3.5 50.16,23.24 49.53,22.61 43.31,22.61 40.64,25.27 40.15,25.27 RN2.6
N$111
  Top 0.254: IC3.10 43.43,23.24 40.64,26.04 40.19,26.04 RN2.7
N$112
  Top 0.254: IC3.6 50.16,24.51 49.15,23.5 48.26,23.5 47.88,23.88 43.56,23.88 40.51,26.93 RN2.8
N$113
  Top 0.254: RN4.16 37.97,36.57 37.47,36.07 35.18,36.07 DP3.7
N$114
  Top 0.254: RN4.15 38.07,37.37 37.34,38.1 32.64,38.1 DP3.8
N$115
  Top 0.254: RN4.14 38.03,38.17 37.59,38.61 30.61,38.61 DP3.9
N$116
  Top 0.254: RN4.13 37.99,38.97 37.85,39.12 28.57,39.12 DP3.10
N$117
  Top 0.254: RN4.12 31.48,39.77 DP3.2
N$118
  Top 0.254: RN4.11 33.22,40.57 DP3.3
N$119
  Top 0.254: RN4.10 37.56,41.37 37.34,41.15 35.18,41.15 DP3.4
N$120
  Top 0.254: RN4.9 DP3.5
N$122
  Top 0.254: RN4.1 40.63,36.57 43.81,39.75 IC5.13
N$123
  Top 0.254: RN4.2 40.67,37.37 43.69,40.39 49.53,40.39 50.16,41.02 IC5.3
N$124
  Top 0.254: RN4.3 40.71,38.17 43.56,41.02 IC5.12
N$125
  Top 0.254: RN4.4 40.75,38.97 43.43,41.66 49.53,41.66 50.16,42.29 IC5.4
N$126
  Top 0.254: RN4.5 40.79,39.77 43.31,42.29 IC5.11
N$127
  Top 0.254: RN4.6 40.82,40.57 43.18,42.93 49.53,42.93 50.16,43.56 IC5.5
N$128
  Top 0.254: RN4.7 40.86,41.37 43.05,43.56 IC5.10
N$129
  Top 0.254: RN4.8 40.9,42.17 42.93,44.2 47.37,44.2 47.75,43.81 49.15,43.81 50.16,44.83 IC5.6
RESET1
  Top 0.254: IC1.1 11.43,44.7 11.3,44.83 8.38,44.83 8.26,44.7 8.26,41.91 6.99,40.64 6.99,34.29 7.62,33.66 JP1.5
RF_IN
  Top 0.254: IC2.2 43.3,8.52 43.31,8.51 44.58,8.51
  Top 0.61: 44.58,8.51 45.85,8.51
  Top 2.007: 45.85,8.51 BU1.SIGNAL
RF_OUT
  Top 0.254: IC2.14 39.38,8.52 39.37,8.51 37.97,8.51
  Top 0.61: 36.7,8.51 37.97,8.51
  Top 2.007: BU2.SIGNAL 36.7,8.51
SCK  (via drill 0.6)
  Top 0.254: 7.75,23.37 10.41,23.37 11.05,24 11.12,24 R5.1
  Top 0.406: IC1.7 JP1.3 10.16,30.48 11.43,29.21 R5.1 | 7.75,23.37 3.68,23.37 3.43,23.62 3.43,46.1 3.68,46.35 v39.62,46.35
  Bottom 0.406: v39.62,46.35 42.04,46.35 43.69,44.7 45.73,44.7 S1.4 S1.3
